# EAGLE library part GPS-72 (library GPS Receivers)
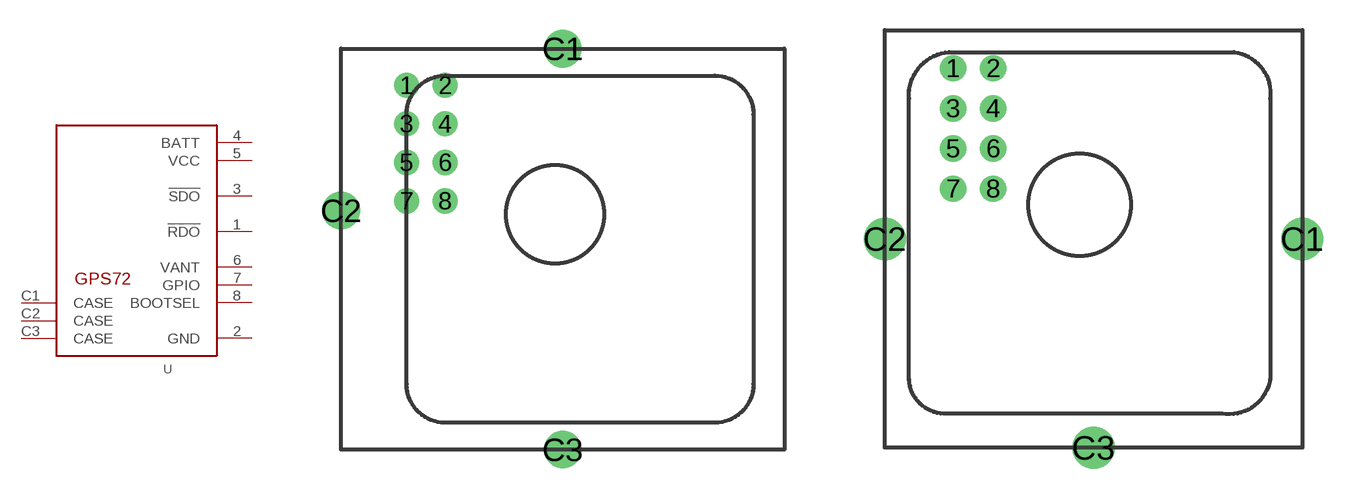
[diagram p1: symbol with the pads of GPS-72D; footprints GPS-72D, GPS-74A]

Designator prefix U

## GPS-72GPS-72D  [GPS-72D]
1  !RDO  in
2  GND  pwr
3  !SDO  out
4  BATT  pwr
5  VCC  pwr
6  VANT  nc
7  GPIO  nc
8  BOOTSEL  nc
C1  CASE
C2  CASE
C3  CASE

## GPS-72GPS-74A  [GPS-74A]
Pads as for GPS-72D

## Footprint GPS-72D (pad centres in mm)
GPS-72D (Position's GPS receiver)
drill 0.8: 1 -8.1,8.5; 2 -6.1,8.5; 3 -8.1,6.5; 4 -6.1,6.5; 5 -8.1,4.5; 6 -6.1,4.5; 7 -8.1,2.5; 8 -6.1,2.5
drill 1.3: C1 0,10.4; C2 -11.5,2; C3 0,-10.4

## Footprint GPS-74A (pad centres in mm)
drill 0.8: 1 -7,8.5; 2 -5,8.5; 3 -7,6.5; 4 -5,6.5; 5 -7,4.5; 6 -5,4.5; 7 -7,2.5; 8 -5,2.5
drill 1.4: C1 10.4,0; C2 -10.4,0; C3 0,-10.4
